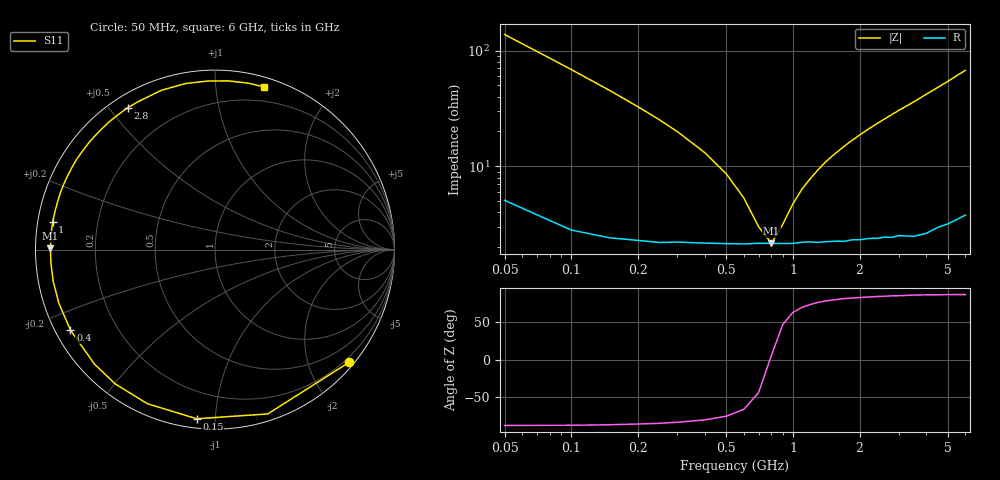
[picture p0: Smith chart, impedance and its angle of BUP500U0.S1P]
! Infineon Technologies  Discrete & RF Semiconductors
! BB 833
! Si Tuning Diode in SOD323
! VR = 0.5 V
! S-Parameters:  June  1999
# GHz  S  MA  R  50
!  f  S11
! GHz  MAG  ANG
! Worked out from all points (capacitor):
!   34 points, 50 MHz to 6 GHz, reference 50 ohm
!   read as one part to ground: C = 22.9 pF near 50 MHz
!   lowest |Z| = 2.17 ohm at 800 MHz (marker M1)
!   series resonance near 790.6 MHz, so ESL is about 1.8 nH
!   S11 on the Smith chart (normalised r, x): 50 MHz: 0.10, -2.75; 150 MHz: 0.05, -0.90; 400 MHz: 0.04, -0.26; 1 GHz: 0.04, +0.08; 2.8 GHz: 0.05, +0.56; 6 GHz: 0.08, +1.35
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0.05  0.9766 -39.9
0.1  0.9616 -72.2
0.15  0.948 -96.2
0.2  0.9377 -113.7
0.25  0.9321 -126.6
0.3  0.9262 -136.5
0.4  0.9217 -150.9
0.5  0.9197 -161.0
0.6  0.9187 -168.8
0.7  0.9172 -175.2
0.8  0.9172 179.5
1  0.9178 170.3
1.1  0.9165 166.3
1.3  0.9182 159.3
1.5  0.9185 152.9
1.6  0.919 150.1
1.8  0.9199 144.4
2  0.9215 139.3
2.2  0.9221 134.4
2.4  0.9245 129.9
2.8  0.9284 121.5
3  0.9288 117.5
3.5  0.9365 108.6
4  0.9399 100.0
4.5  0.94 92.3
5  0.943 85.4
5.5  0.9454 78.7
6  0.9475 73.1
